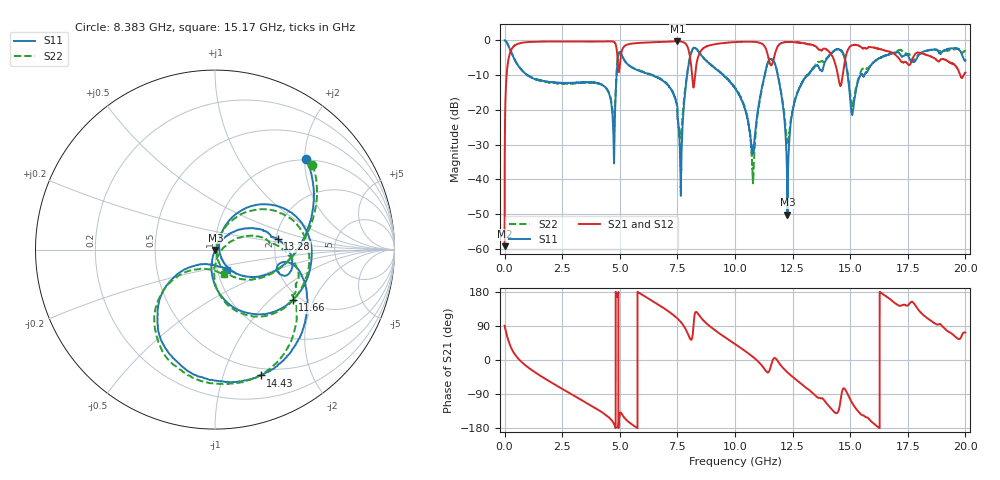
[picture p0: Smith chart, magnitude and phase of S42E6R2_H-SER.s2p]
!{S42E6R2}
!Johanson Technology Inc.
!www.johansontechnology.com
!Test Board Conditions:
!Substrate Type  RO4350B
!Substrate Thickness  50 mil
!Substrate Dk  3.66
!TL Type: GCPW
!TL Trace Width  60 mil
!TL Gap  10 mil
!Electrode orientation  Horizontal
!DUT TOPOLOGY	SERIES
!Mounting Pad LxW  14x55 mil
! Created Wed Nov 25 21:48:39 2020
# khz S ma R 50
! 2 Port Network Data from SP1.SP block
! freq  magS11  angS11  magS21  angS21  magS12  angS12  magS22  angS22
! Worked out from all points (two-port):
!   20001 points, 300 kHz to 20 GHz, reference 50 ohm
!   highest |S21| = -0.23 dB at 7.502 GHz (marker M1); lowest = -59.2 dB at 300 kHz (marker M2)
!   |S21| within 3 dB of the highest: 254.4 MHz to 4.877 GHz (4.622 GHz wide, 180 % of centre); 5.08 GHz to 8.005 GHz (2.925 GHz wide, 44.7 % of centre)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
!   lowest |S11| = -50.2 dB at 12.28 GHz (marker M3), VSWR 1.01, Z = 50.3 - j0.16 ohm
!   |S11| at or under -10 dB: 992.6 MHz to 4.859 GHz (3.866 GHz wide, 132 % of centre); 6.392 GHz to 7.921 GHz (1.53 GHz wide, 21.4 % of centre); 9.499 GHz to 11.28 GHz (1.783 GHz wide, 17.2 % of centre)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
!   |S22| runs from -41.1 to 0.0 dB; largest |S21 - S12| = 0.019
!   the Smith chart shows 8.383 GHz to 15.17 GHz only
!   S11 on the Smith chart (normalised r, x): 8.383 GHz: 0.98, +2.03; 11.66 GHz: 1.82, -1.40; 13.28 GHz: 2.05, +0.28; 14.43 GHz: 0.42, -1.34; 15.17 GHz: 1.11, -0.26
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300  0.9992 -0.3  0.001095 90.5  0.001139 90.5  0.9971 -0.1
113300  0.9149 -27.7  0.3983 62.0  0.3996 61.9  0.9148 -27.8
326300  0.6307 -63.0  0.7714 27.2  0.7728 27.1  0.6328 -63.2
1740300  0.2595 -137.5  0.9641 -48.7  0.9647 -48.8  0.2562 -139.6
3334300  0.2491 161.3  0.9658 -105.4  0.9643 -105.4  0.2452 167.5
4711300  0.0568 111.1  0.9635 -164.5  0.9639 -164.5  0.07992 148.0
5005300  0.6782 161.0  0.4577 -141.0  0.4588 -141.2  0.688 157.3
6667300  0.2883 58.9  0.9485 146.2  0.9472 146.1  0.2928 55.8
7502300  0.08077 24.8  0.9734 109.4  0.9721 109.5  0.07983 35.8
7666300  0.01393 162.4  0.9631 98.8  0.9629 99.0  0.0484 117.3
8018300  0.5074 131.6  0.6581 60.0  0.6579 59.8  0.5211 120.5
8383300  0.7166 44.8  0.5571 123.0  0.5542 122.9  0.7202 41.0
1.00003e7  0.2055 -44.5  0.9469 42.1  0.9498 42.2  0.211 -50.4
1.07843e7  0.02455 18.1  0.9553 7.8  0.9559 7.9  0.009279 -5.8
1.16633e7  0.5163 -33.2  0.5156 2.5  0.5155 2.7  0.5113 -37.2
1.22773e7  0.003104 -30.8  0.9502 -32.6  0.9511 -32.7  0.0335 -40.2
1.32763e7  0.3547 9.7  0.8764 -82.1  0.8773 -81.8  0.3609 2.0
1.33343e7  0.3726 6.6  0.8643 -85.2  0.8679 -85.0  0.3843 -0.3
1.44333e7  0.7457 -70.0  0.3579 -139.9  0.3625 -139.9  0.7496 -75.0
1.51683e7  0.1317 -59.5  0.8613 -120.9  0.8687 -121.2  0.1477 -70.2
1.66673e7  0.6248 -104.2  0.6961 163.6  0.6807 163.5  0.6268 -114.4
2e7  0.5148 139.2  0.3458 72.5  0.3481 73.1  0.7057 133.9
